(* Logix 5000 AddOnInstructionDefinition export; software revision 16.04 *)

ADD_ON_INSTRUCTION AMCI_ANG1E_Configure   (* revision 1.0 *)
VAR_INPUT
   slot_axis_number : INT; {required}   // 0=all switches off 1=switch 1 on 2=switch 2 on 3=switch 3 on 4=switch 4 on 5=swich 5 on
   Input_1_Function : INT; {required}
   Input_1_Active_State : BOOL; {required}
   Input_2_Function : INT; {required}
   Input_2_Active_State : BOOL; {required}
   Input_3_Function : INT; {required}
   Input_3_Active_State : BOOL; {required}
   Z_Input_Home : BOOL;
   Encoder_Enable : BOOL; {required}
   Backplane_Home_Proximity_Enable : BOOL;
   Stall_Detect_Enable : BOOL;
   Antiresonance : BOOL;
   Input_Data_Format_0_standard_1_binary : BOOL;
   Output_State_Network_Lost : BOOL;
   Output_Control_Network_Lost : BOOL;
   Output_Functionality : BOOL;
   Drive_Enable : BOOL;
   Starting_Speed : DINT; {required}
   Motor_Steps_Turn : INT; {required}
   Encoder_Counts_Turn : INT; {required}
   Idle_Current : INT; {required}
   Motor_Current : INT; {required}
   Current_Loop_Gain : INT; {required}
END_VAR
VAR_IN_OUT
   AMCI_ANG1E_Output_data : INT[10]; {required}
END_VAR
VAR
   upper_result_X_1000 : DINT;
   command_data_block : INT[10];
        [0].15   // Mode Bit 1=Configuraiton Mode 0=Command Mode
   index : INT;
END_VAR

ROUTINE Logic   (* ladder *)
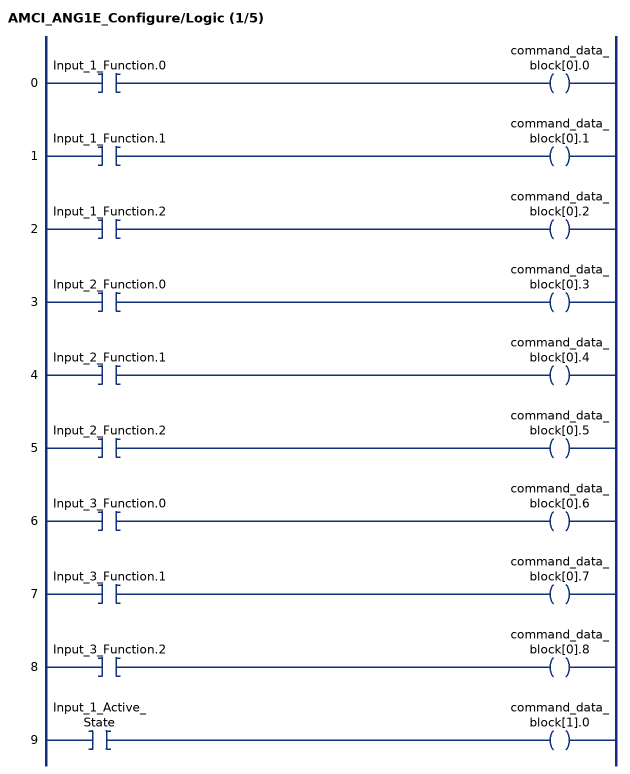
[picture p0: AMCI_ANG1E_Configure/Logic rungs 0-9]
   0: XIC(Input_1_Function.0)OTE(command_data_block[0].0);
   1: XIC(Input_1_Function.1)OTE(command_data_block[0].1);
   2: XIC(Input_1_Function.2)OTE(command_data_block[0].2);
   3: XIC(Input_2_Function.0)OTE(command_data_block[0].3);
   4: XIC(Input_2_Function.1)OTE(command_data_block[0].4);
   5: XIC(Input_2_Function.2)OTE(command_data_block[0].5);
   6: XIC(Input_3_Function.0)OTE(command_data_block[0].6);
   7: XIC(Input_3_Function.1)OTE(command_data_block[0].7);
   8: XIC(Input_3_Function.2)OTE(command_data_block[0].8);
   9: XIC(Input_1_Active_State)OTE(command_data_block[1].0);
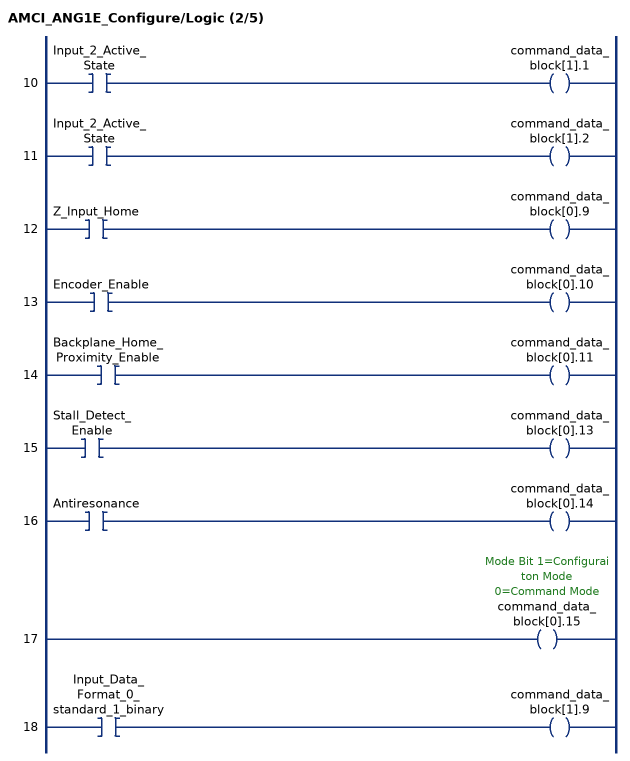
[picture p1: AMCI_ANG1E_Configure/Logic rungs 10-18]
   10: XIC(Input_2_Active_State)OTE(command_data_block[1].1);
   11: XIC(Input_2_Active_State)OTE(command_data_block[1].2);
   12: XIC(Z_Input_Home)OTE(command_data_block[0].9);
   13: XIC(Encoder_Enable)OTE(command_data_block[0].10);
   14: XIC(Backplane_Home_Proximity_Enable)OTE(command_data_block[0].11);
   15: XIC(Stall_Detect_Enable)OTE(command_data_block[0].13);
   16: XIC(Antiresonance)OTE(command_data_block[0].14);
   17: OTE(command_data_block[0].15);
   18: XIC(Input_Data_Format_0_standard_1_binary)OTE(command_data_block[1].9);
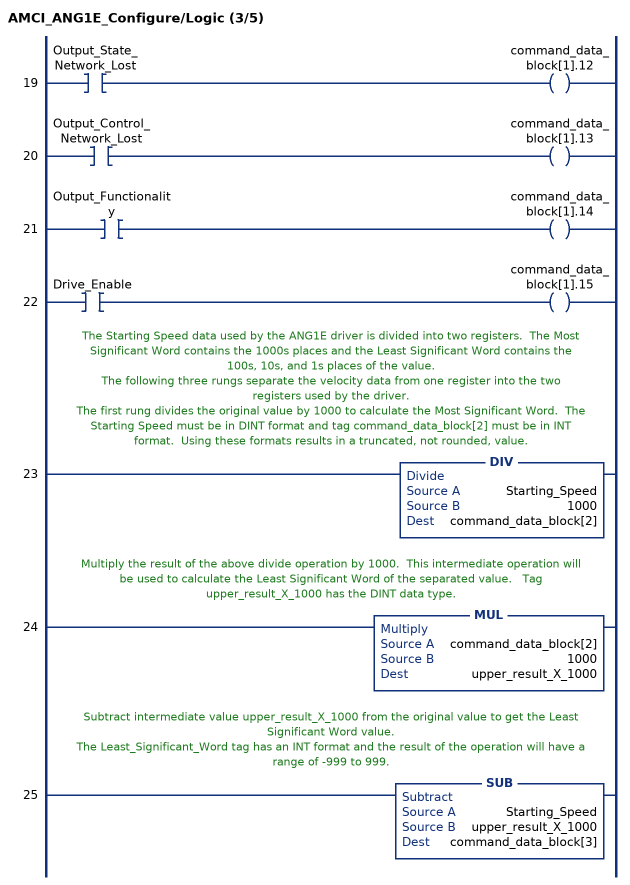
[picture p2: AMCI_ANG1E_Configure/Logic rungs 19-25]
   19: XIC(Output_State_Network_Lost)OTE(command_data_block[1].12);
   20: XIC(Output_Control_Network_Lost)OTE(command_data_block[1].13);
   21: XIC(Output_Functionality)OTE(command_data_block[1].14);
   22: XIC(Drive_Enable)OTE(command_data_block[1].15);
   // The Starting Speed data used by the ANG1E driver is divided into two registers.  The Most Significant Word contains the 1000s places and the Least Significant Word contains the 100s, 10s, and 1s places of the value.
   // The following three rungs separate the velocity data from one register into the two registers used by the driver.
   // The first rung divides the original value by 1000 to calculate the Most Significant Word.  The Starting Speed must be in DINT format and tag command_data_block[2] must be in INT format.  Using these formats results in a truncated, not rounded, value.
   23: DIV(Starting_Speed,1000,command_data_block[2]);
   // Multiply the result of the above divide operation by 1000.  This intermediate operation will be used to calculate the Least Significant Word of the separated value.   Tag upper_result_X_1000 has the DINT data type.
   24: MUL(command_data_block[2],1000,upper_result_X_1000);
   // Subtract intermediate value upper_result_X_1000 from the original value to get the Least Significant Word value.
   // The Least_Significant_Word tag has an INT format and the result of the operation will have a range of -999 to 999.
   25: SUB(Starting_Speed,upper_result_X_1000,command_data_block[3]);
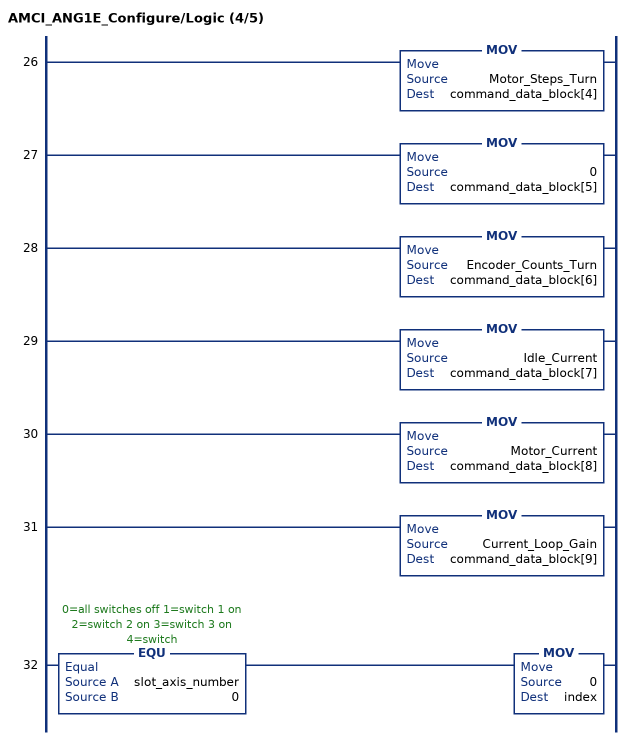
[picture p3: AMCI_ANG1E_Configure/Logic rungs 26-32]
   26: MOV(Motor_Steps_Turn,command_data_block[4]);
   27: MOV(0,command_data_block[5]);
   28: MOV(Encoder_Counts_Turn,command_data_block[6]);
   29: MOV(Idle_Current,command_data_block[7]);
   30: MOV(Motor_Current,command_data_block[8]);
   31: MOV(Current_Loop_Gain,command_data_block[9]);
   32: EQU(slot_axis_number,0)MOV(0,index);
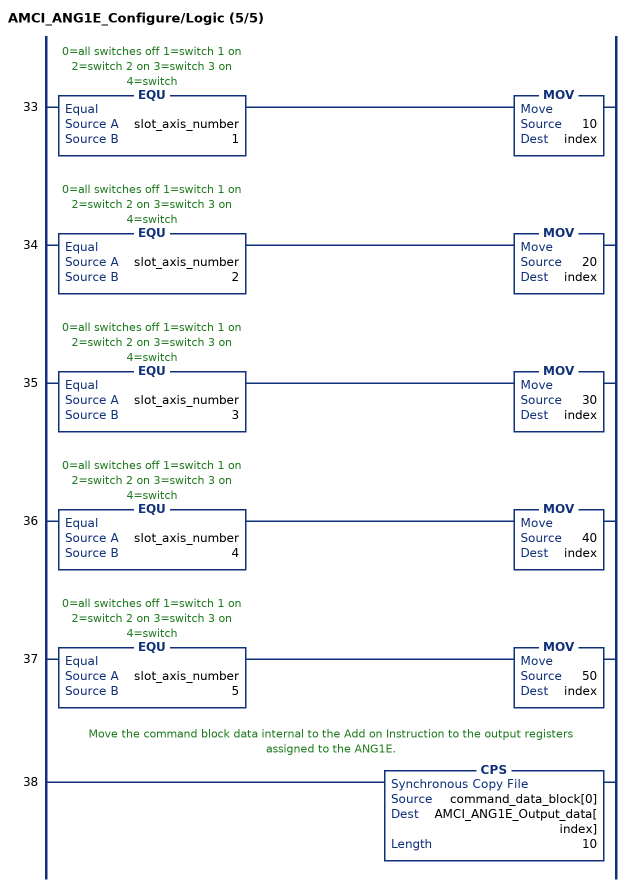
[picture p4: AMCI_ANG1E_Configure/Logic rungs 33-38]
   33: EQU(slot_axis_number,1)MOV(10,index);
   34: EQU(slot_axis_number,2)MOV(20,index);
   35: EQU(slot_axis_number,3)MOV(30,index);
   36: EQU(slot_axis_number,4)MOV(40,index);
   37: EQU(slot_axis_number,5)MOV(50,index);
   // Move the command block data internal to the Add on Instruction to the output registers assigned to the ANG1E.
   38: CPS(command_data_block[0],AMCI_ANG1E_Output_data[index],10);
END_ROUTINE
END_ADD_ON_INSTRUCTION
